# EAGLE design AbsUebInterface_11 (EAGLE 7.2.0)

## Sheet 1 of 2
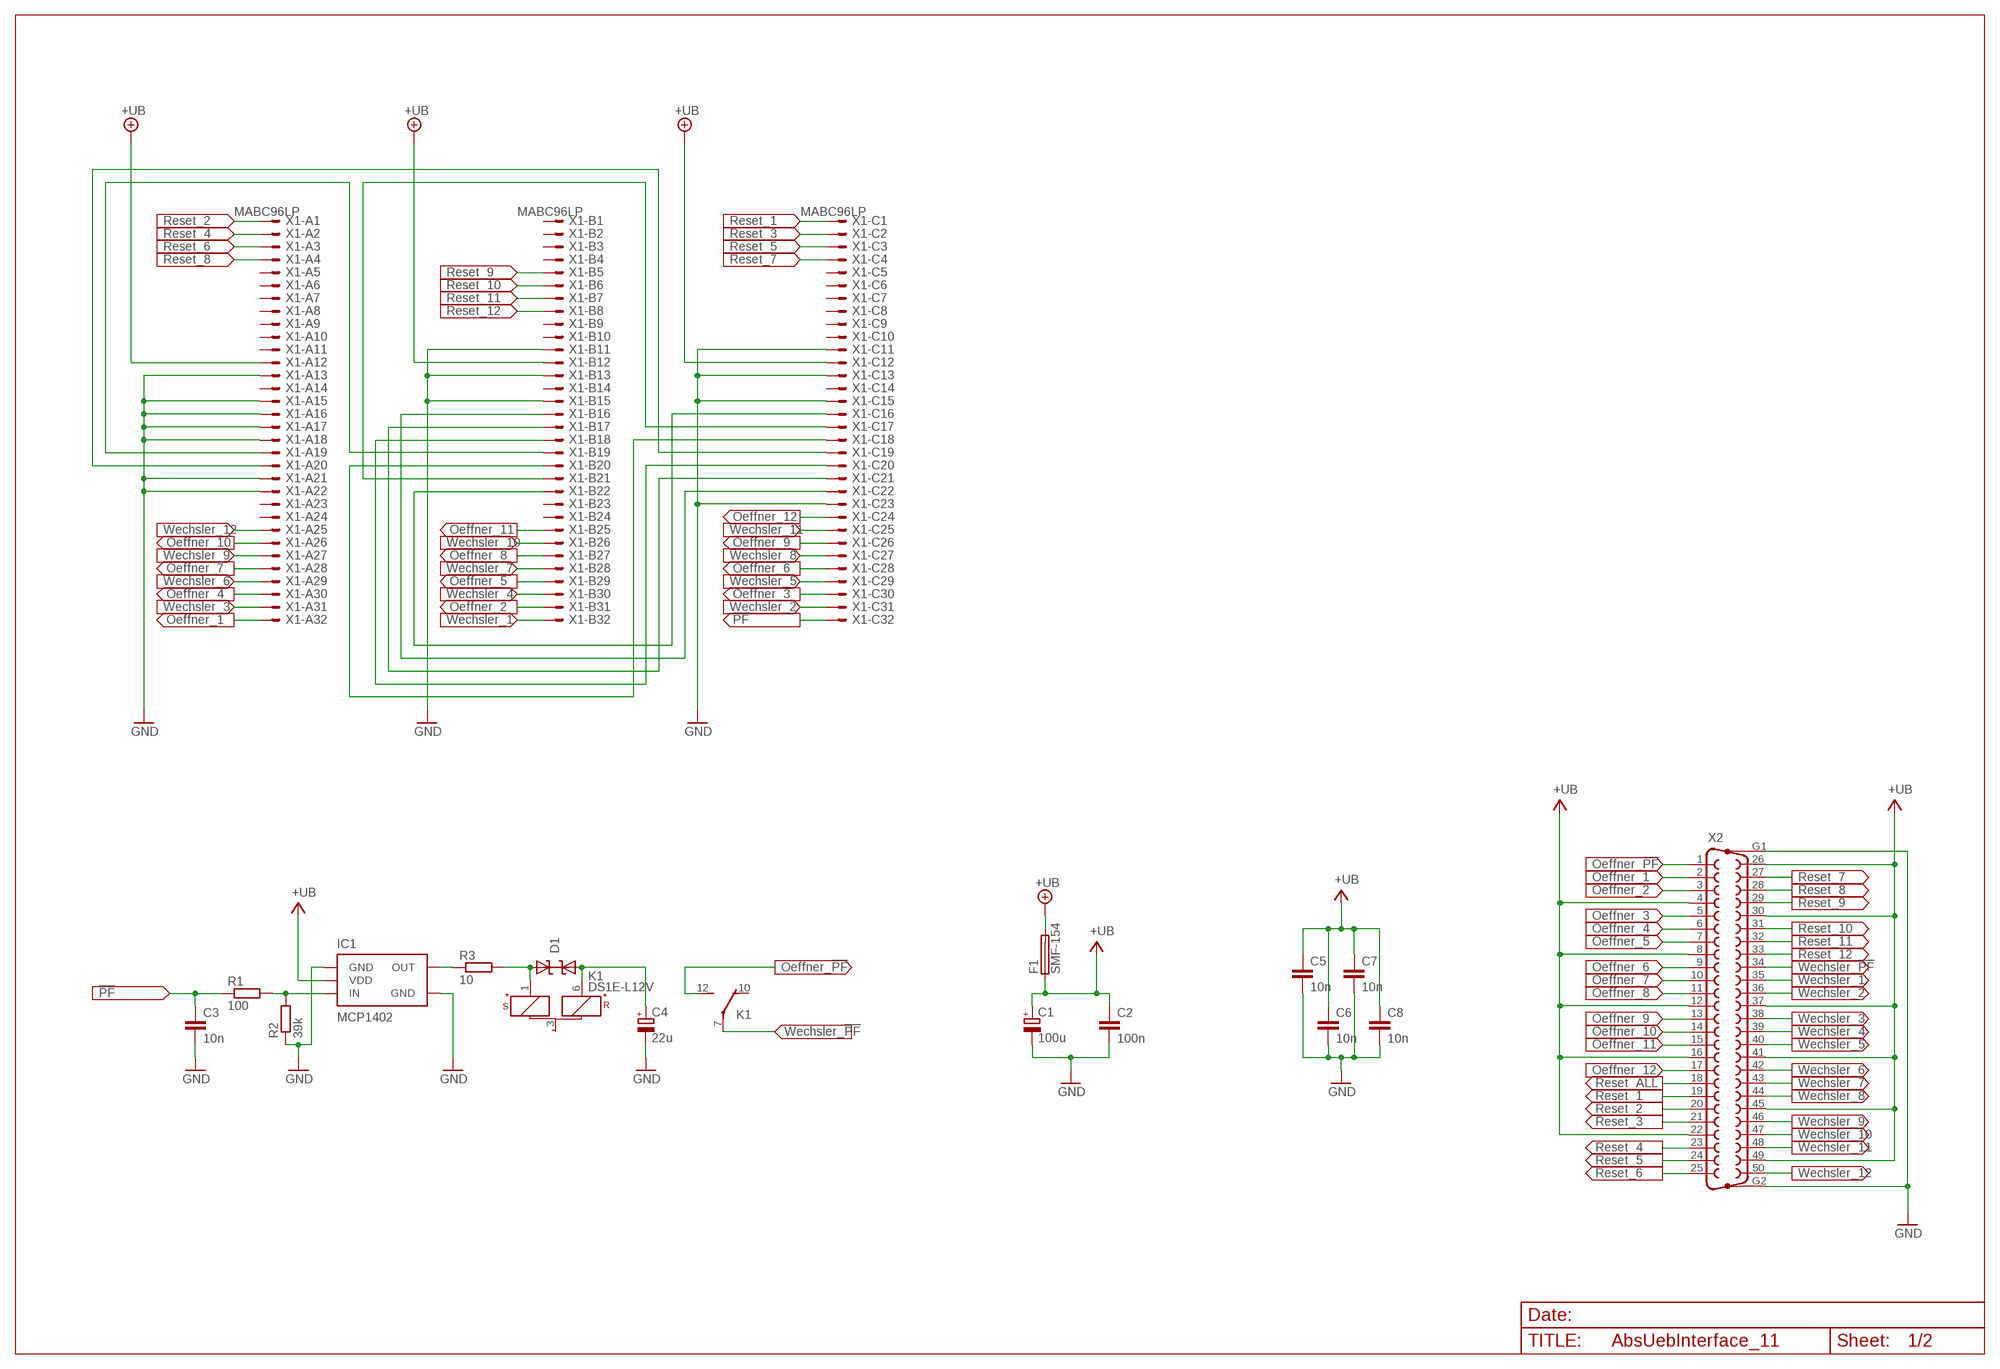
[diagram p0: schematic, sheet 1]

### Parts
C1  100u  CPOL-5-10  [RAD-FR-5,0-10]
C2  100n  C-SMD-1206  [C1206]
C3  10n  C-SMD-1206  [C1206]
C4  22u  CPOL-2-5  [RAD-FR-2,0-5]
C5  10n  C-SMD-1206  [C1206]
C6  10n  C-SMD-1206  [C1206]
C7  10n  C-SMD-1206  [C1206]
C8  10n  C-SMD-1206  [C1206]
D1  P6SMB11CAT3  [SMB-DO-214AA]
F1  SMF-154  [SMF-154]
IC1  MCP1402  [SOT223-5]
K1  DS1E-L12V  [DS1E-L]
R1  100  R-SMD-1206  [R1206]
R2  39k  R-SMD-1206  [R1206]
R3  10  R-SMD-1206  [R1206]
X1  MABC96LP  [MABC96LP]
X2  F50HP  [F50HP]

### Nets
1-WIRE: X1.B21 X1.C17
!PF: C3.1 R1.1 X1.C32
+UB: F1.2 X1.A12 X1.B12 X1.C12
CANH: X1.B16 X1.C22
CANL: X1.B22 X1.C16
EXT_PNP: X1.A20 X1.C19
EXT_RESET: X1.A19 X1.B19
GND: C1.- C2.2 C3.2 C4.- C5.2 C6.2 C7.2 C8.2 IC1.1(GND) IC1.4(GND) R2.1 X1.A13 X1.A15 X1.A16 X1.A17 X1.A18 X1.A21 X1.A22 X1.B11 X1.B13 X1.B15 X1.C11 X1.C13 X1.C15 X1.C23 X2.G1 X2.G2 ; also sheet 2
N$1: IC1.5(OUT) R3.1
N$2: D1.1(C) K1.1(1:S+) R3.2
N$3: IC1.3(IN) R1.2 R2.2
N$4: C4.+ D1.2(A) K1.6(1:R+)
N$5: X1.B20 X1.C18
OEFFNER_1: X1.A32 X2.2
OEFFNER_2: X1.B31 X2.3
OEFFNER_3: X1.C30 X2.5
OEFFNER_4: X1.A30 X2.6
OEFFNER_5: X1.B29 X2.7
OEFFNER_6: X1.C28 X2.9
OEFFNER_7: X1.A28 X2.10
OEFFNER_8: X1.B27 X2.11
OEFFNER_9: X1.C26 X2.13
OEFFNER_10: X1.A26 X2.14
OEFFNER_11: X1.B25 X2.15
OEFFNER_12: X1.C24 X2.17
OEFFNER_!PF: K1.12(2:S) X2.1
RESET_1: X1.C1 X2.19 ; also sheet 2
RESET_2: X1.A1 X2.20 ; also sheet 2
RESET_3: X1.C2 X2.21 ; also sheet 2
RESET_4: X1.A2 X2.23 ; also sheet 2
RESET_5: X1.C3 X2.24 ; also sheet 2
RESET_6: X1.A3 X2.25 ; also sheet 2
RESET_7: X1.C4 X2.27 ; also sheet 2
RESET_8: X1.A4 X2.28 ; also sheet 2
RESET_9: X1.B5 X2.29 ; also sheet 2
RESET_10: X1.B6 X2.31 ; also sheet 2
RESET_11: X1.B7 X2.32 ; also sheet 2
RESET_12: X1.B8 X2.33 ; also sheet 2
RESET_ALL: X2.18 ; also sheet 2
SCL: X1.B18 X1.C20
SDA: X1.B17 X1.C21
V+: C1.+ C2.1 C5.1 C6.1 C7.1 C8.1 F1.1 IC1.2(VDD) X2.4 X2.8 X2.12 X2.16 X2.22 X2.26 X2.30 X2.37 X2.41 X2.45 X2.49 ; supply symbol labelled +UB ; also sheet 2
WECHSLER_1: X1.B32 X2.35
WECHSLER_2: X1.C31 X2.36
WECHSLER_3: X1.A31 X2.38
WECHSLER_4: X1.B30 X2.39
WECHSLER_5: X1.C29 X2.40
WECHSLER_6: X1.A29 X2.42
WECHSLER_7: X1.B28 X2.43
WECHSLER_8: X1.C27 X2.44
WECHSLER_9: X1.A27 X2.46
WECHSLER_10: X1.B26 X2.47
WECHSLER_11: X1.C25 X2.48
WECHSLER_12: X1.A25 X2.50
WECHSLER_!PF: K1.7(2:P) X2.34
Unconnected: K1.3(1:-) K1.10(2:O) X1.A5 X1.A6 X1.A7 X1.A8 X1.A9 X1.A10 X1.A11 X1.A14 X1.A23 X1.A24 X1.B1 X1.B2 X1.B3 X1.B4 X1.B9 X1.B10 X1.B14 X1.B23 X1.B24 X1.C5 X1.C6 X1.C7 X1.C8 X1.C9 X1.C10 X1.C14

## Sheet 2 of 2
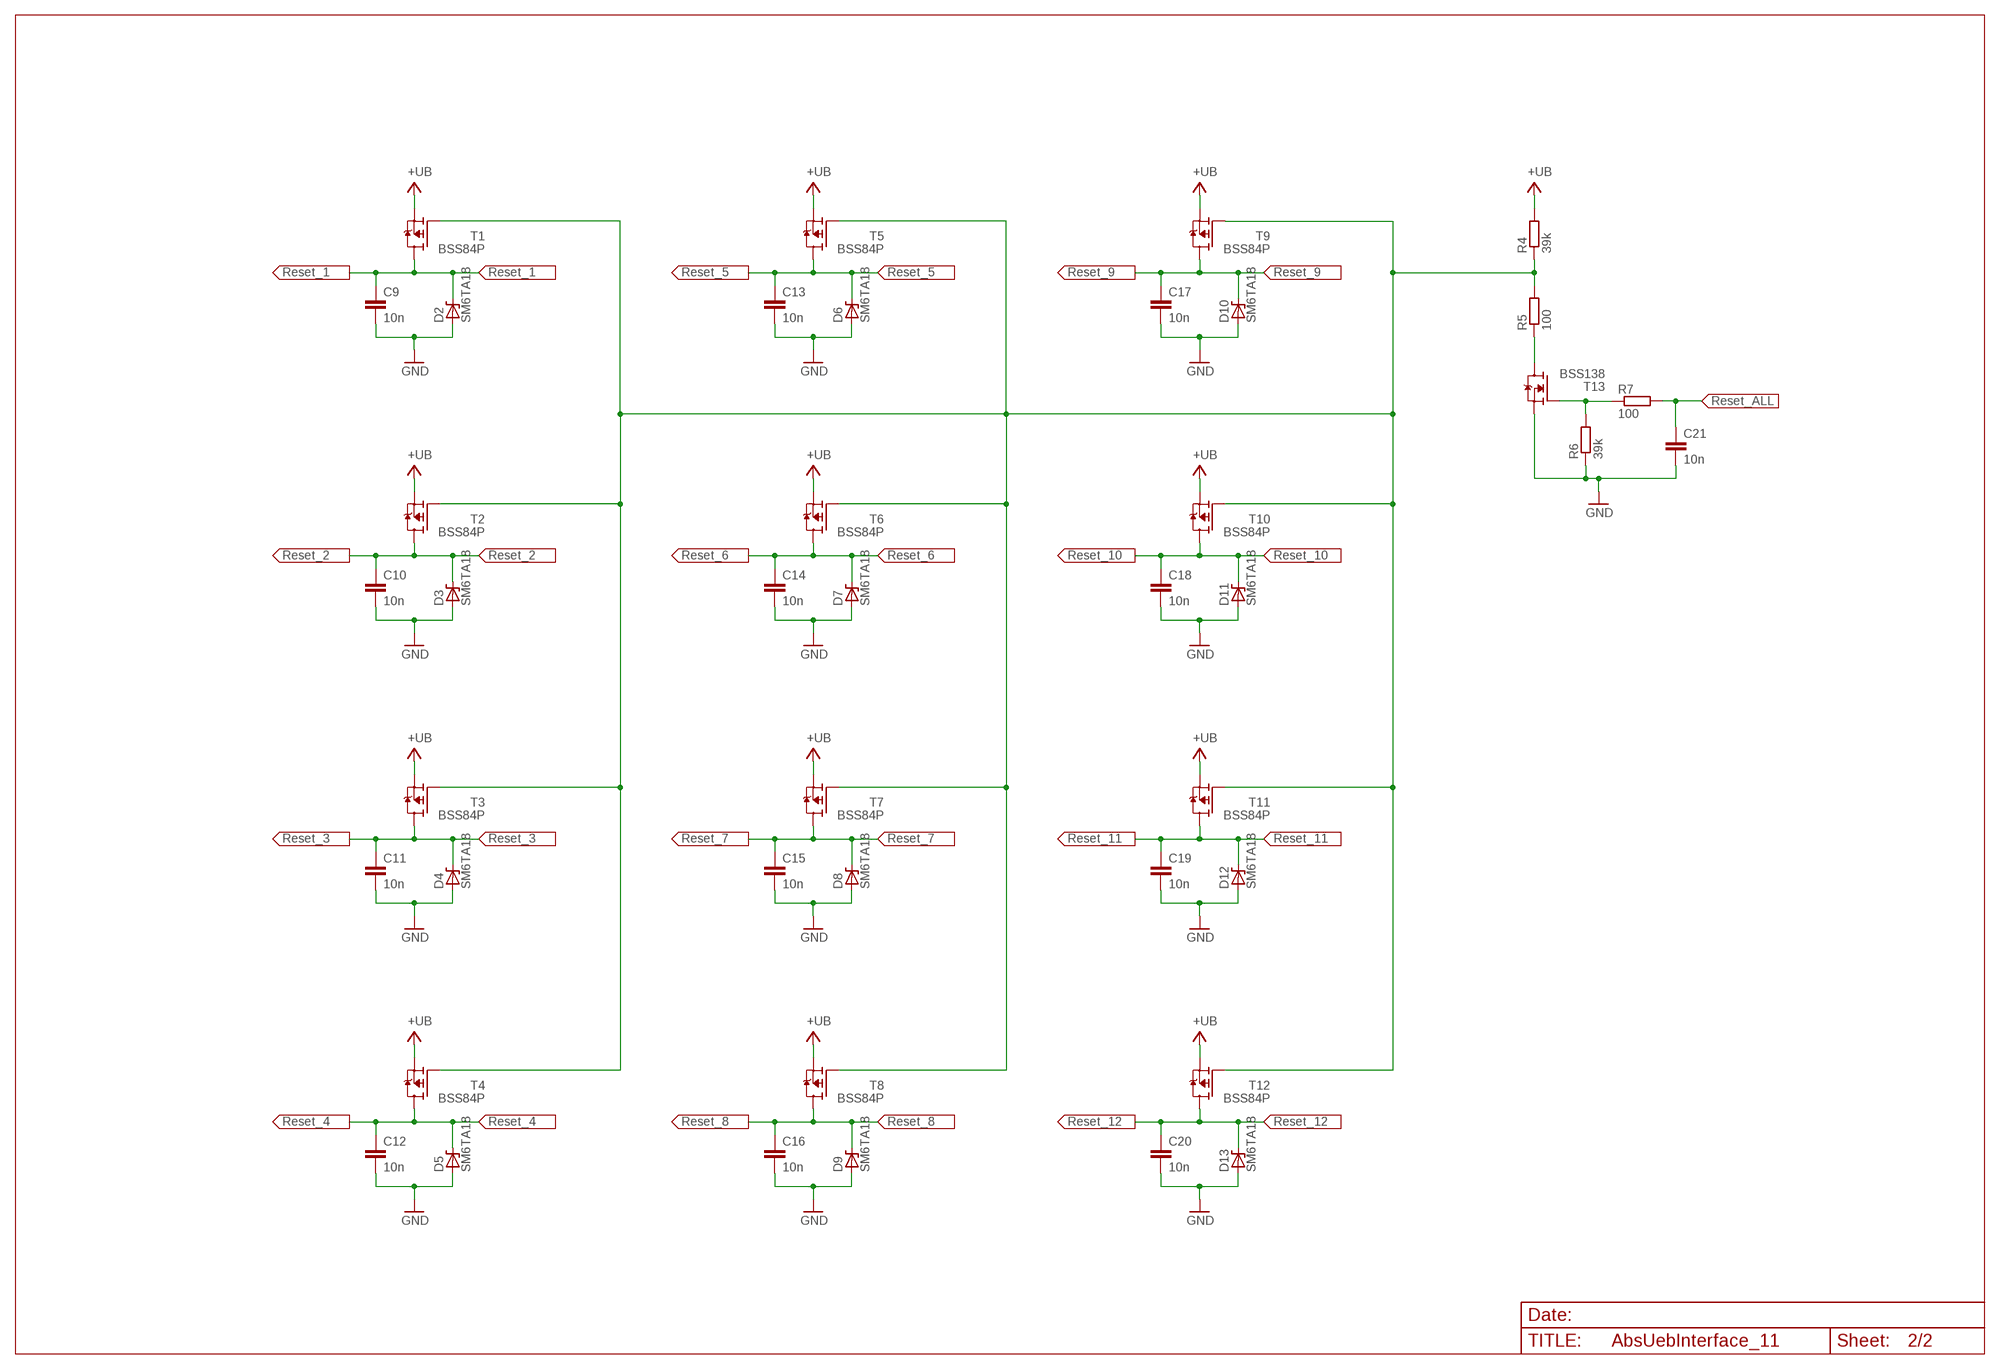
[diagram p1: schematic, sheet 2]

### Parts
C9  10n  C-SMD-1206  [C1206]
C10  10n  C-SMD-1206  [C1206]
C11  10n  C-SMD-1206  [C1206]
C12  10n  C-SMD-1206  [C1206]
C13  10n  C-SMD-1206  [C1206]
C14  10n  C-SMD-1206  [C1206]
C15  10n  C-SMD-1206  [C1206]
C16  10n  C-SMD-1206  [C1206]
C17  10n  C-SMD-1206  [C1206]
C18  10n  C-SMD-1206  [C1206]
C19  10n  C-SMD-1206  [C1206]
C20  10n  C-SMD-1206  [C1206]
C21  10n  C-SMD-1206  [C1206]
D2  SM6TA18  [DO-214AA]
D3  SM6TA18  [DO-214AA]
D4  SM6TA18  [DO-214AA]
D5  SM6TA18  [DO-214AA]
D6  SM6TA18  [DO-214AA]
D7  SM6TA18  [DO-214AA]
D8  SM6TA18  [DO-214AA]
D9  SM6TA18  [DO-214AA]
D10  SM6TA18  [DO-214AA]
D11  SM6TA18  [DO-214AA]
D12  SM6TA18  [DO-214AA]
D13  SM6TA18  [DO-214AA]
R4  39k  R-SMD-1206  [R1206]
R5  100  R-SMD-1206  [R1206]
R6  39k  R-SMD-1206  [R1206]
R7  100  R-SMD-1206  [R1206]
T1  BSS84P  [SOT23]
T2  BSS84P  [SOT23]
T3  BSS84P  [SOT23]
T4  BSS84P  [SOT23]
T5  BSS84P  [SOT23]
T6  BSS84P  [SOT23]
T7  BSS84P  [SOT23]
T8  BSS84P  [SOT23]
T9  BSS84P  [SOT23]
T10  BSS84P  [SOT23]
T11  BSS84P  [SOT23]
T12  BSS84P  [SOT23]
T13  BSS138  [SOT23]

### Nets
GND: C9.2 C10.2 C11.2 C12.2 C13.2 C14.2 C15.2 C16.2 C17.2 C18.2 C19.2 C20.2 C21.2 D2.1(A) D3.1(A) D4.1(A) D5.1(A) D6.1(A) D7.1(A) D8.1(A) D9.1(A) D10.1(A) D11.1(A) D12.1(A) D13.1(A) R6.1 T13.2(S) ; also sheet 1
N$6: R6.2 R7.1 T13.1(G)
N$7: R5.1 T13.3(D)
N$8: R4.1 R5.2 T1.1(G) T2.1(G) T3.1(G) T4.1(G) T5.1(G) T6.1(G) T7.1(G) T8.1(G) T9.1(G) T10.1(G) T11.1(G) T12.1(G)
RESET_1: C9.1 D2.2(C) T1.3(D) ; also sheet 1
RESET_2: C10.1 D3.2(C) T2.3(D) ; also sheet 1
RESET_3: C11.1 D4.2(C) T3.3(D) ; also sheet 1
RESET_4: C12.1 D5.2(C) T4.3(D) ; also sheet 1
RESET_5: C13.1 D6.2(C) T5.3(D) ; also sheet 1
RESET_6: C14.1 D7.2(C) T6.3(D) ; also sheet 1
RESET_7: C15.1 D8.2(C) T7.3(D) ; also sheet 1
RESET_8: C16.1 D9.2(C) T8.3(D) ; also sheet 1
RESET_9: C17.1 D10.2(C) T9.3(D) ; also sheet 1
RESET_10: C18.1 D11.2(C) T10.3(D) ; also sheet 1
RESET_11: C19.1 D12.2(C) T11.3(D) ; also sheet 1
RESET_12: C20.1 D13.2(C) T12.3(D) ; also sheet 1
RESET_ALL: C21.1 R7.2 ; also sheet 1
V+: R4.2 T1.2(S) T2.2(S) T3.2(S) T4.2(S) T5.2(S) T6.2(S) T7.2(S) T8.2(S) T9.2(S) T10.2(S) T11.2(S) T12.2(S) ; supply symbol labelled +UB ; also sheet 1

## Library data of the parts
C1 = AbsUebParts_11:CPOL-5-10: Elektrolytkondensator RM 5,0mm; MF: Panasonic; OC_REICHELT: RAD FR 100/63
C2 C3 C5-C21 = AbsUebParts_11:C-SMD: SMD Keramik Vielschichtkondensatoren
C4 = AbsUebParts_11:CPOL-2-5: Elektrolytkondensator RM 2,0mm; MF: Panasonic; OC_REICHELT: RAD FR 22/50
D1 = AbsUebParts_11:P6SMB11CAT3: Suppressor diode bi-directional
D2-D13 = AbsUebParts_11:SM6TA: STM Transil Suppressor Diode; MF: STM; MPN: SM6T18A; OC_REICHELT: P6SMB 18A SMD
F1 = AbsUebParts_11:SMF-154: Littelfuse Surface Mount Fuse; MF: Littelfuse; MPN: 154.250; OC_REICHELT: SMD-HASF 0,25A; OC_RS: 219-6068
IC1 = AbsUebParts_11:MCP1402: MCP1402 500mA. High-Speed Power MOSFET Driver; MF: Microchip; MPN: MCP1402; OC_RS: 668-4203
K1 = AbsUebParts_11:DS1E-L*: DS-RELAYS HIGHLY SENSITIVE 1500 V FCC SURGE NAiS WITHSTANDING MINIATURE RELAY Source: http://www.mew-europe.com/.. en_ds_61005_0001.pdf; MF: Panasonic; MPN: DS2E-SL2-DC12V; OC_RS: 815-4988
R1-R7 = AbsUebParts_11:R-SMD: SMD Resistor
T1-T12 = AbsUebParts_11:BSS84P: Infineon SIPMOS P-Channel Small-Signal-Transistor; MF: Infineon; MPN: BSS 84 P; OC_REICHELT: BSS 84P SMD
T13 = AbsUebParts_11:BSS138: Infineon NFET N-Channel Logic Level Enhancement Mode Field Effect Transistor; MF: FSC; MPN: BSS138; OC_REICHELT: BSS 138 SMD
X1 = AbsUebParts_11:MABC96LP: CONNECTOR male, 96 pins, type C, rows ABC, grid 2.54 mm with mounting clip; MF: ept; OC_REICHELT: ML-C 96W
X2 = AbsUebParts_11:F50HP: SUB-D; MF: CONEC; MPN: 164A18759X; OC_FARNELL: unknown; OC_REICHELT: D-SUB BU 50GWC

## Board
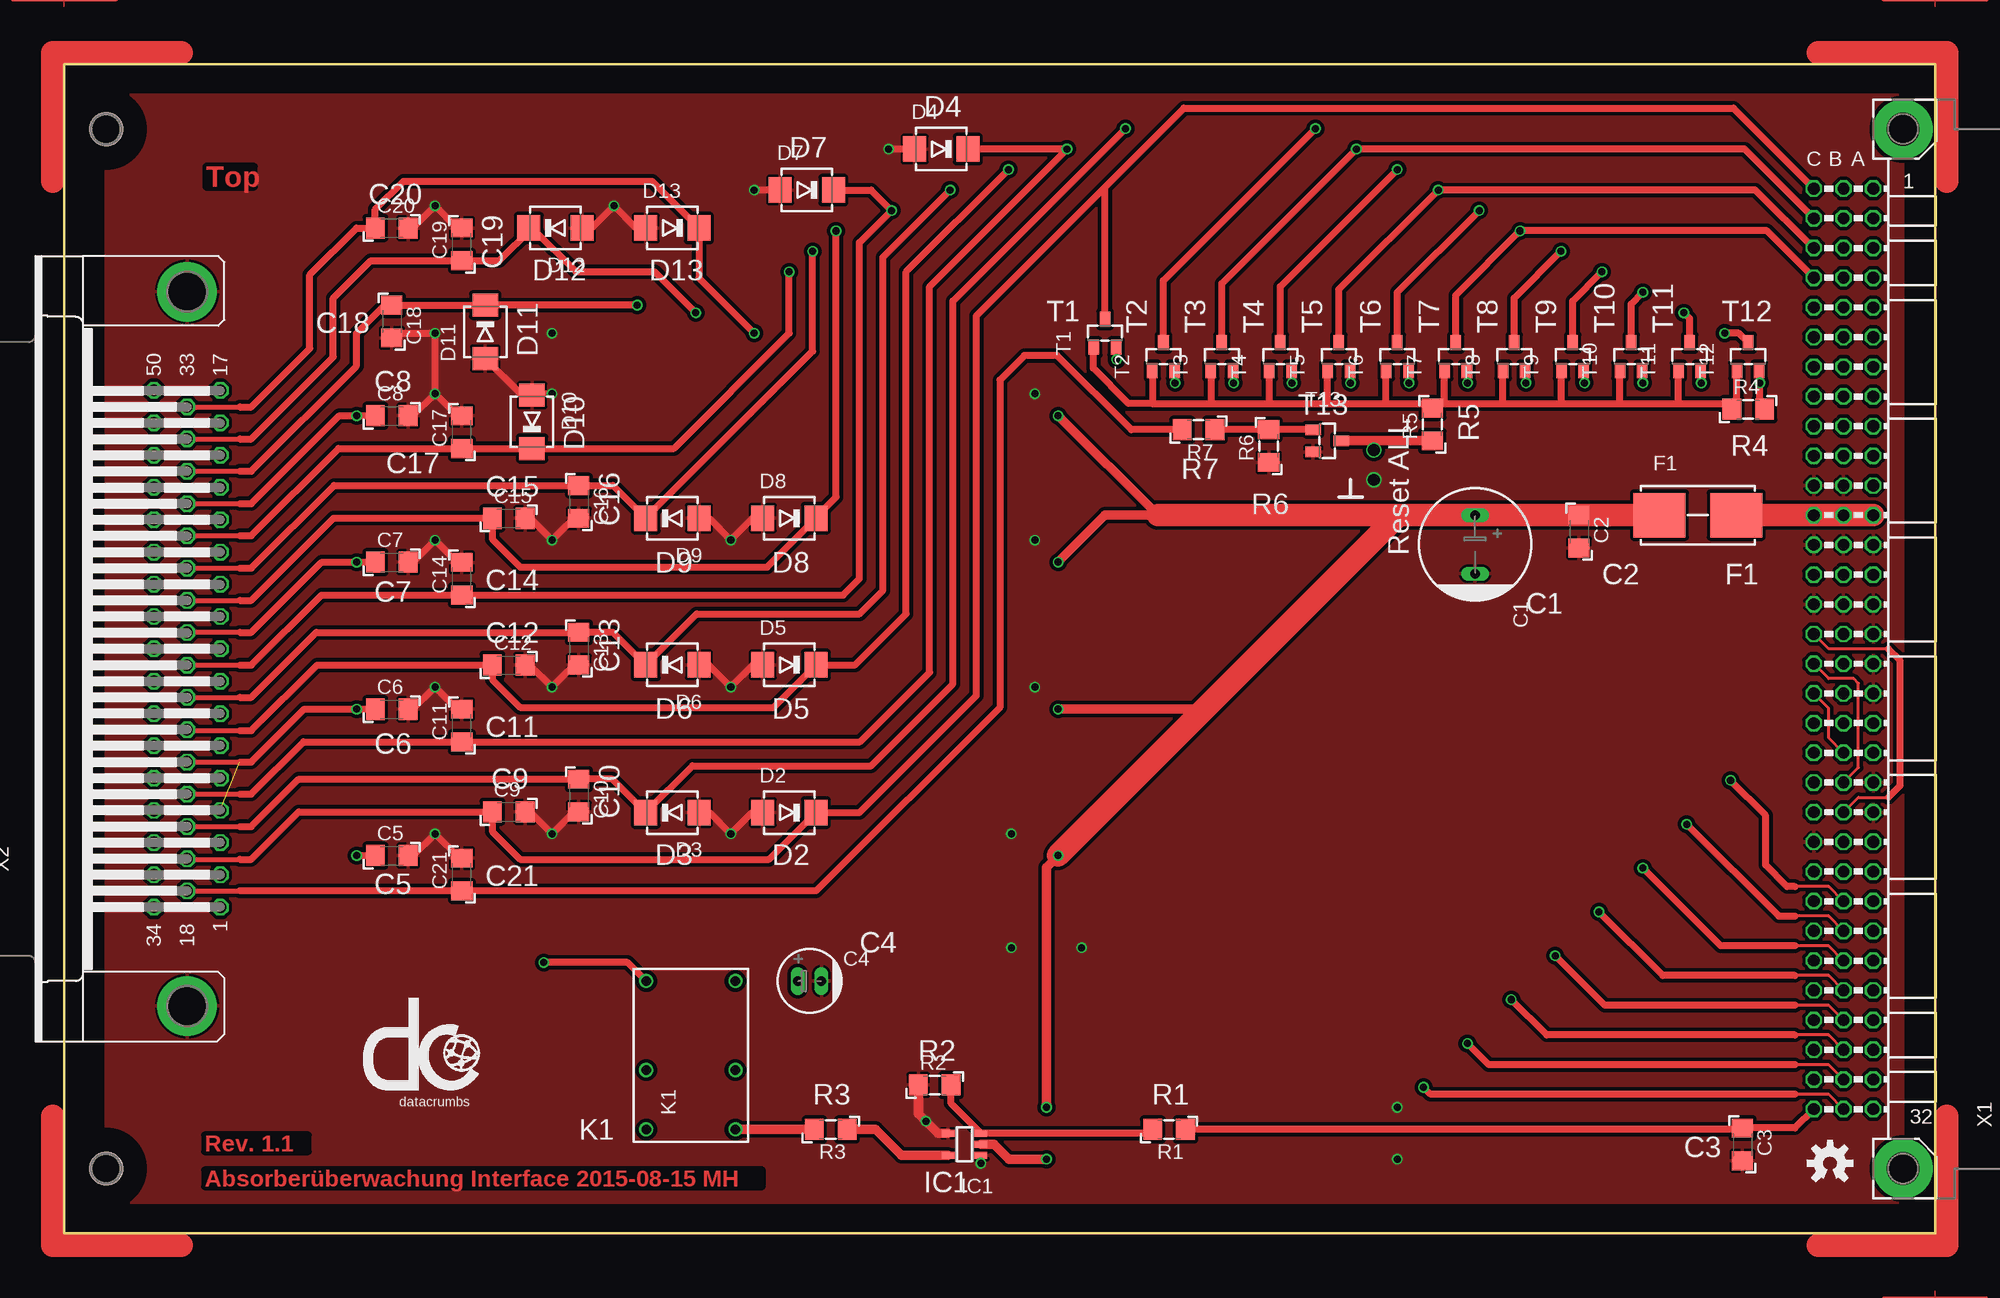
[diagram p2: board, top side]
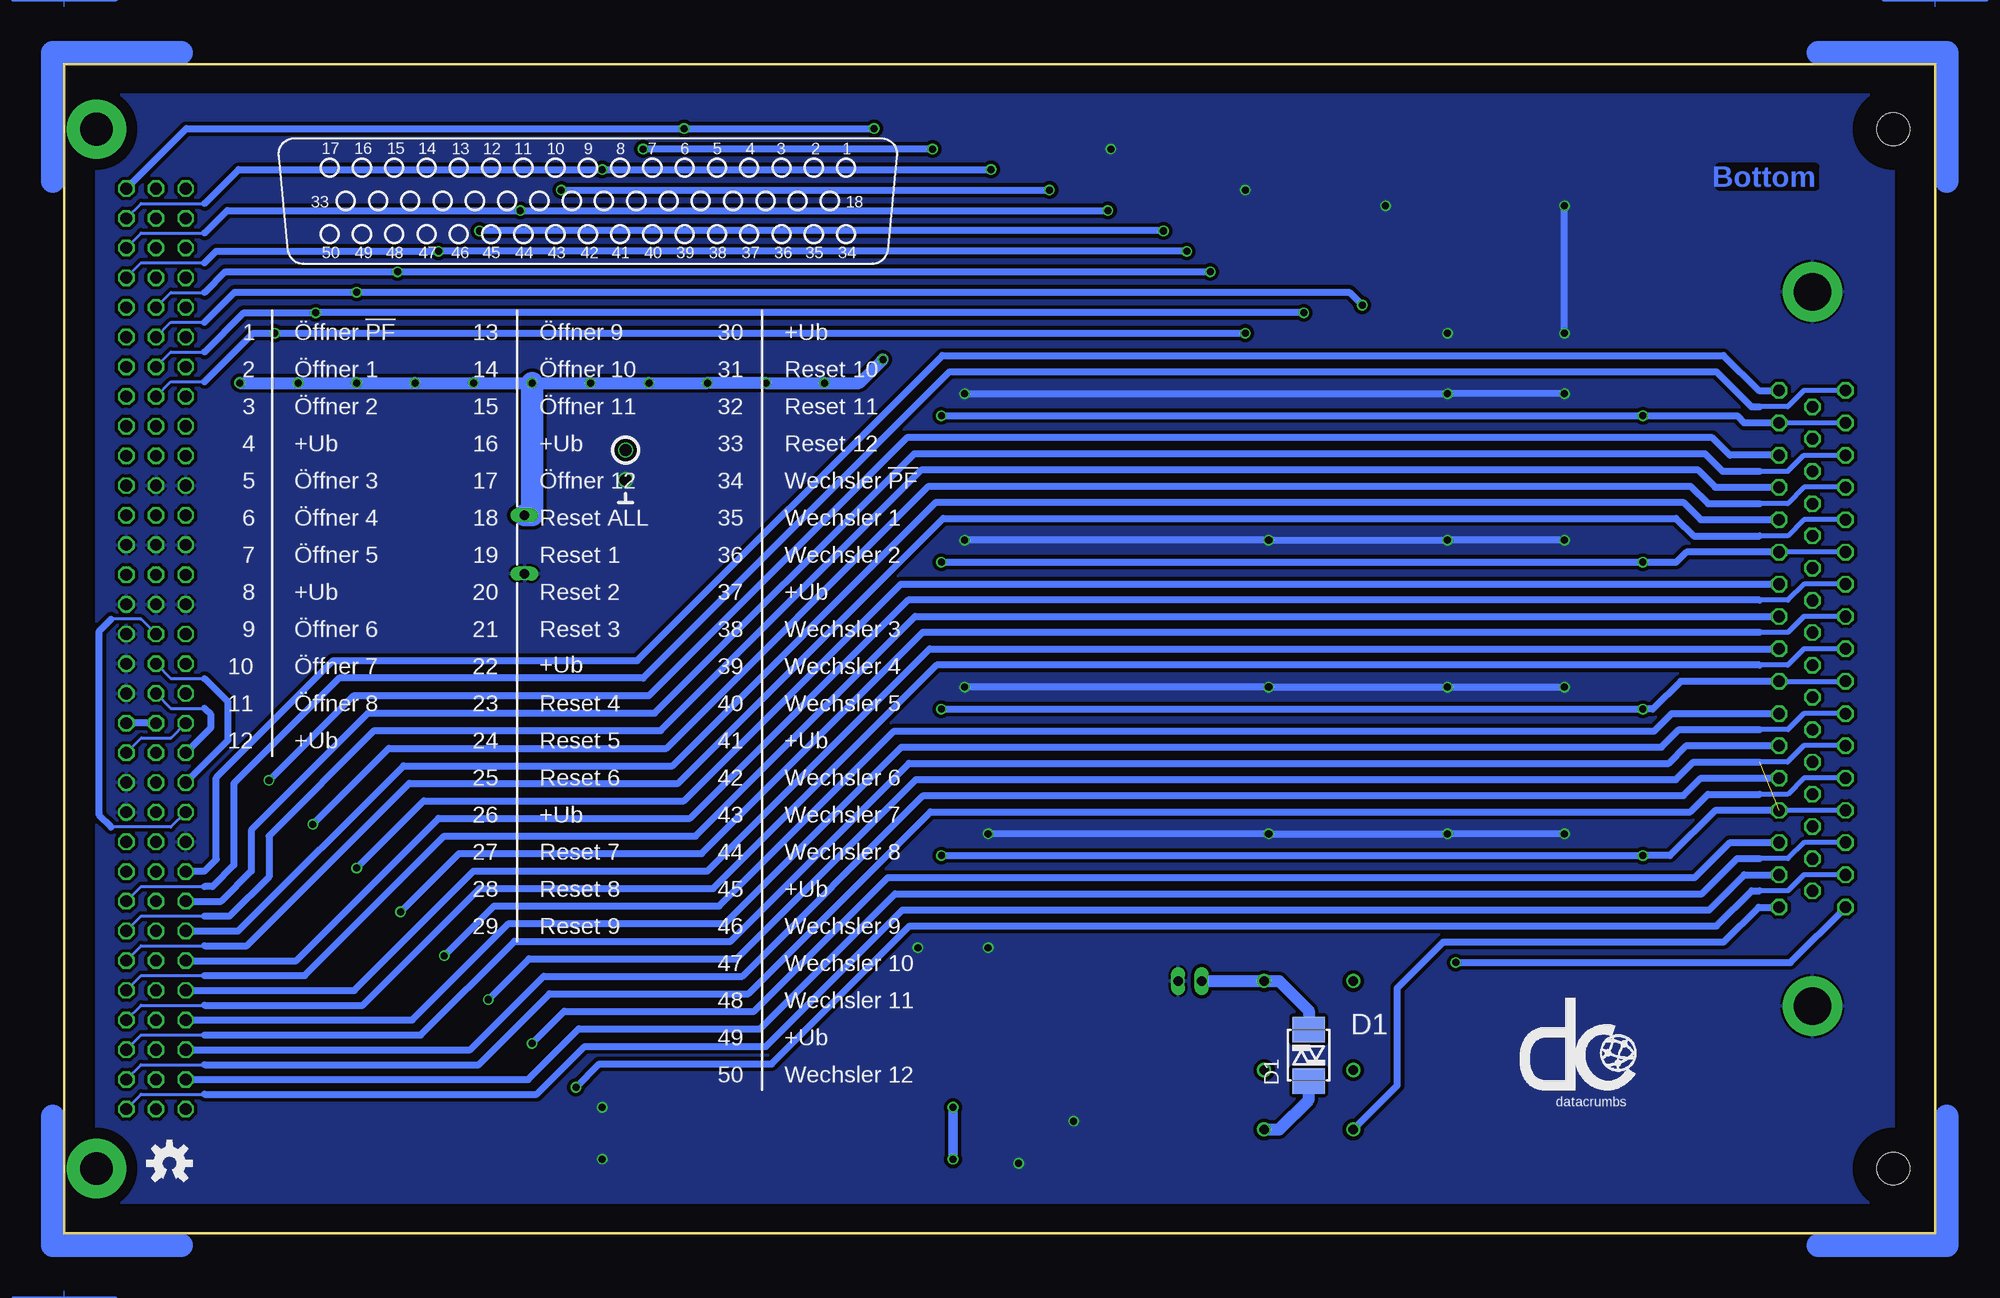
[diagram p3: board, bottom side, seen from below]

Size 160.03 x 100.03 mm. Coordinates in mm from the lower left corner, seen from the top.
Outline: 0,0.01 160,0.01 160,100.01 0,100.01 0,0.01
Copper layers (1*16): Top 0.035mm / dielectric 1.5mm / Bottom 0.035mm
Design rules "Aetzwerk-DRC 2 Lagen 35µm Cu *": minimum track width 6mil, minimum drill 12mil, track to track 6mil, track to pad 6mil, pad to pad 6mil, via to via 6mil, smd to smd 6mil, copper to edge 20mil, drill to drill 8mil, minimum pad ring 8mil, minimum via ring 6mil, stop-mask expansion 3mil, vias tented up to drill 24mil, thermal gap 8mil
Holes 2.8 mm at 3.57,94.46 3.57,5.56
tKeepout: area 0,0 to 160,2.5; area 0,97.5 to 160,100
bKeepout: area 0,0 to 160,2.5; area 0,97.5 to 160,100
tRestrict: area 1.3,92.2 to 5.9,96.7; area 1.3,3.3 to 5.9,7.8
bRestrict: area 1.3,92.2 to 5.9,96.7; area 1.3,3.3 to 5.9,7.8
vRestrict: area 1.3,3.3 to 5.9,7.8; area 1.3,92.2 to 5.9,96.7

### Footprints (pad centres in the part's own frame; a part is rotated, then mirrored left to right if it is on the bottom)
RAD-FR-5,0-10 = drill 0.8 long: + -2.5,0; - 2.5,0
C1206 = smd 1.6 x 1.8: 1 -1.4,0; 2 1.4,0
RAD-FR-2,0-5 = drill 0.8 long: + -1,0; - 1,0
SMB-DO-214AA = smd 2.16 x 2.75: 1 -2.2,0; 2 2.2,0
DO-214AA = smd 1.96 x 2.18: 1 -2.28,0; 2 2.28,0
SMF-154 = smd 4.445 x 3.81: 1 -3.289,0; 2 3.289,0
SOT223-5 = smd 0.6 x 1.1: 1 -0.95,-1.4; 2 0,-1.4; 3 0.95,-1.4; 4 0.95,1.4; 5 -0.95,1.4
DS1E-L = drill 0.8: 1 -6.35,-3.81; 3 -1.27,-3.81; 6 6.35,-3.81; 7 6.35,3.81; 10 -1.27,3.81; 12 -6.35,3.81
R1206 = smd 1.6 x 1.8: 1 -1.4,0; 2 1.4,0
SOT23 = smd 0.9 x 1.3: 1 -0.95,-1.2; 2 0.95,-1.2; 3 0,1.2
MABC96LP = drill 1 octagon: A1 -2.54,39.37; A2 -2.54,36.83; A3 -2.54,34.29; A4 -2.54,31.75; A5 -2.54,29.21; A6 -2.54,26.67; A7 -2.54,24.13; A8 -2.54,21.59; A9 -2.54,19.05; A10 -2.54,16.51; A11 -2.54,13.97; A12 -2.54,11.43; A13 -2.54,8.89; A14 -2.54,6.35; A15 -2.54,3.81; A16 -2.54,1.27; A17 -2.54,-1.27; A18 -2.54,-3.81; A19 -2.54,-6.35; A20 -2.54,-8.89; A21 -2.54,-11.43; A22 -2.54,-13.97; A23 -2.54,-16.51; A24 -2.54,-19.05; A25 -2.54,-21.59; A26 -2.54,-24.13; A27 -2.54,-26.67; A28 -2.54,-29.21; A29 -2.54,-31.75; A30 -2.54,-34.29; A31 -2.54,-36.83; A32 -2.54,-39.37; B1 -5.08,39.37; B2 -5.08,36.83; B3 -5.08,34.29; B4 -5.08,31.75; B5 -5.08,29.21; B6 -5.08,26.67; B7 -5.08,24.13; B8 -5.08,21.59; B9 -5.08,19.05; B10 -5.08,16.51; B11 -5.08,13.97; B12 -5.08,11.43; B13 -5.08,8.89; B14 -5.08,6.35; B15 -5.08,3.81; B16 -5.08,1.27; B17 -5.08,-1.27; B18 -5.08,-3.81; B19 -5.08,-6.35; B20 -5.08,-8.89; B21 -5.08,-11.43; B22 -5.08,-13.97; B23 -5.08,-16.51; B24 -5.08,-19.05; B25 -5.08,-21.59; B26 -5.08,-24.13; B27 -5.08,-26.67; B28 -5.08,-29.21; B29 -5.08,-31.75; B30 -5.08,-34.29; B31 -5.08,-36.83; B32 -5.08,-39.37; C1 -7.62,39.37; C2 -7.62,36.83; C3 -7.62,34.29; C4 -7.62,31.75; C5 -7.62,29.21; C6 -7.62,26.67; C7 -7.62,24.13; C8 -7.62,21.59; C9 -7.62,19.05; C10 -7.62,16.51; C11 -7.62,13.97; C12 -7.62,11.43; C13 -7.62,8.89; C14 -7.62,6.35; C15 -7.62,3.81; C16 -7.62,1.27; C17 -7.62,-1.27; C18 -7.62,-3.81; C19 -7.62,-6.35; C20 -7.62,-8.89; C21 -7.62,-11.43; C22 -7.62,-13.97; C23 -7.62,-16.51; C24 -7.62,-19.05; C25 -7.62,-21.59; C26 -7.62,-24.13; C27 -7.62,-26.67; C28 -7.62,-29.21; C29 -7.62,-31.75; C30 -7.62,-34.29; C31 -7.62,-36.83; C32 -7.62,-39.37 | drill 2.8 pad 5.08: X1 0,44.45; X2 0,-44.45
F50HP = drill 1 octagon: 1 -22.1,-2.84; 2 -19.33,-2.84; 3 -16.56,-2.84; 4 -13.82,-2.84; 5 -11.05,-2.84; 6 -8.28,-2.84; 7 -5.54,-2.84; 8 -2.77,-2.84; 9 0,-2.84; 10 2.77,-2.84; 11 5.54,-2.84; 12 8.28,-2.84; 13 11.05,-2.84; 14 13.82,-2.84; 15 16.56,-2.84; 16 19.33,-2.84; 17 22.1,-2.84; 18 -20.7,0; 19 -17.96,0; 20 -15.19,0; 21 -12.42,0; 22 -9.68,0; 23 -6.91,0; 24 -4.14,0; 25 -1.4,0; 26 1.4,0; 27 4.14,0; 28 6.91,0; 29 9.68,0; 30 12.42,0; 31 15.19,0; 32 17.96,0; 33 20.7,0; 34 -22.1,2.84; 35 -19.33,2.84; 36 -16.56,2.84; 37 -13.82,2.84; 38 -11.05,2.84; 39 -8.28,2.84; 40 -5.54,2.84; 41 -2.77,2.84; 42 0,2.84; 43 2.77,2.84; 44 5.54,2.84; 45 8.28,2.84; 46 11.05,2.84; 47 13.82,2.84; 48 16.56,2.84; 49 19.33,2.84; 50 22.1,2.84 | drill 3.2 pad 5.08: G1 -30.55,0; G2 30.55,0

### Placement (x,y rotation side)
C1  120.65,58.94 270 top
C2  129.54,60.04 270 top
C3  143.51,7.63 270 top
C4  63.74,21.6 0 top
C5  28,32.33 0 top
C6  28,44.85 0 top
C7  28,57.42 0 top
C8  28,69.95 0 top
C9  38,36.07 0 top
C10  44,37.47 270 top
C11  34,43.45 90 top
C12  38,48.63 0 top
C13  44,50.03 270 top
C14  34,56.01 90 top
C15  38,61.18 0 top
C16  44,62.58 270 top
C17  34,68.55 90 top
C18  28,78.01 270 top
C19  34,84.61 90 top
C20  28,86.01 0 top
C21  34,30.71 90 top
D1  53.58,15.25 90 bottom
D2  62,36.01 0 top
D3  52,36.01 180 top
D4  75,92.76 0 top
D5  62,48.64 0 top
D6  52,48.64 180 top
D7  63.5,89.26 0 top
D8  62,61.18 0 top
D9  52,61.18 180 top
D10  40,69.43 270 top
D11  36,77.13 90 top
D12  42,86.01 180 top
D13  52,86.01 0 top
DRILEGEND  [DRILEGEND]  not placed on the board
F1  139.7,61.44 0 top
IC1  76.98,7.63 90 top
K1  53.58,15.25 90 top
PM1  [PASSMARK]  not placed on the board
PM2  [PASSMARK]  not placed on the board
PM3  [PASSMARK]  not placed on the board
R1  94.47,8.9 180 top
R2  74.44,12.71 0 top
R3  65.55,8.9 180 top
R4  144,70.51 0 top
R5  117,69.21 90 top
R6  103,67.36 90 top
R7  97,68.76 180 top
T1  89,77.01 0 top
T2  94,75.01 0 top
T3  99,75.01 0 top
T4  104,75.01 0 top
T5  109,75.01 0 top
T6  114,75.01 0 top
T7  119,75.01 0 top
T8  124,75.01 0 top
T9  129,75.01 0 top
T10  134,75.01 0 top
T11  139,75.01 0 top
T12  144,75.01 0 top
T13  108,67.81 270 top
X1  157.24,50.01 0 top
X2  10.5,50.01 90 top

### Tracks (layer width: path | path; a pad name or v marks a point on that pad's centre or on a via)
1-WIRE
  Top 0.254: X1.B21 153.44,39.86 153.44,47.06 153.02,47.47 150.89,47.47 X1.C17
!PF
  Top 0.61: X1.C32 148.01,9.03 C3.1 143.38,8.9 R1.1
+UB
  Top 1.93: F1.2 X1.C12 X1.B12 X1.A12
CANH
  Bottom 0.254: X1.C22 150.89,34.77 156,34.77 | X1.B16 153.43,52.55 156,52.55
  Bottom 0.61: 156,34.77 157,35.77 157,51.55 156,52.55
CANL
  Top 0.254: X1.B22 153.43,37.31 156,37.31 | 156,50.01 150.89,50.01 X1.C16
  Top 0.61: 156,37.31 157,38.31 157,49.01 156,50.01
CM10
  Top 2: -1,10.01 -1,-0.99 10,-0.99
CM11
  Bottom 2: 10,-0.99 -1,-0.99 -1,10.01
CM20
  Top 2: 150,-0.99 161,-0.99 161,10.01
CM21
  Bottom 2: 150,-0.99 161,-0.99 161,10.01
CM30
  Top 2: 10,101.01 -1,101.01 -1,90.01
CM31
  Bottom 2: -1,90.01 -1,101.01 10,101.01
CM40
  Top 2: 150,101.01 161,101.01 161,90.01
CM41
  Bottom 2: 150,101.01 161,101.01 161,90.01
EXT_PNP
  Bottom 0.254: X1.A20 153.42,42.41 150.88,42.41 X1.C19
EXT_RESET
  Bottom 0.61: X1.B19 X1.A19
GND  (via drill 0.6, 1)
  Top 0.406: v78.38,6.01 IC1.1
  Top 0.61: C15.2 39.82,61.18 v41.7,59.3 43.58,61.18 C16.2 | C12.2 39.81,48.63 v41.7,46.74 43.59,48.63 C13.2 | C9.2 39.83,36.07 v41.7,34.2 43.57,36.07 C10.2 44.06,36.01 | C8.2 29.81,69.95 v31.7,71.84 | C17.2 33.59,69.95 v31.7,71.84 | C7.2 29.82,57.42 v31.7,59.3 33.59,57.41 C14.2 | C6.2 29.81,44.85 v31.7,46.74 33.59,44.85 C11.2 | C19.2 33.59,86.01 v31.7,87.9 29.81,86.01 C20.2 | v31.7,71.84 v31.7,77.01 28.4,77.01 C18.2 | 39.87,71.84 D10.1 40.13,71.84 v41.7,71.84 39.01,71.84 D11.1 | D3.1 55.19,36.01 v57,34.2 58.81,36.01 D2.1 | D6.1 55.1,48.64 v57,46.74 58.9,48.64 D5.1 | D9.1 55.12,61.18 v57,59.3 58.88,61.18 D8.1 | D13.1 48.89,86.01 v47,87.9 45.11,86.01 D12.1 | D7.1 v59,89.26 | D4.1 v70.5,92.76 | 33.79,32.11 v31.7,34.2 29.83,32.33 C5.2
  Top 0.813: IC1.4 74.71,8.58 v73.67,9.61 73.04,10.25 R2.1
  Bottom 0.61: v31.7,34.2 v41.7,34.2 v57,34.2 v81,34.2 | v31.7,59.3 v41.7,59.3 v57,59.3 v83,59.3 | v31.7,46.74 v41.7,46.74 v57,46.74 v83,46.74 | v31.7,77.01 v31.7,87.9 | v31.7,71.84 v41.7,71.84 v83,71.84
  other vias: 114,10.8 114,6.36 81,24.44 41.7,77.01 87,24.44 112,64.47
  pour Top (isolate 0.305): 3.57,2.66 157.24,2.66 157.24,97.36 3.57,97.36
  pour Bottom (isolate 0.305): 3.57,2.66 157.24,2.66 157.24,97.36 3.57,97.36
N$1
  Top 0.813: IC1.5 71.58,6.68 69.36,8.9 R3.1
N$2
  Top 0.813: K1.1 R3.2
  Bottom 1.016: K1.1 56.12,8.9 53.58,11.44 D1.1
N$3
  Top 0.61: R1.2 92.75,8.58 IC1.3 75.84,11.12 R2.2
N$4
  Bottom 1.016: C4.+ K1.6 56.12,21.6 53.58,19.06 D1.2
N$5
  Top 0.254: X1.B20 150.89,42.39 150.89,44.93 X1.C18
N$6
  Top 0.61: T13.1 R6.2 R7.1
N$7  (via drill 1)
  Top 0.813: T13.3 112,67.81 | 112,67.81 R5.1 | v112,67.01 112,67.81
N$8
  Top 0.61: 93,71.01 98,71.01 | 108,71.01 113,71.01 | 118,71.01 123,71.01 | 123,71.01 128,71.01 | 128,71.01 133,71.01 | 133,71.01 138,71.01 | T12.1 143,73.76 143,71.41 R4.1 142.1,71.01 138,71.01 | T2.1 93.05,71.06 93,71.01 | T3.1 98.05,71.06 98,71.01 | T5.1 108,73.81 108,71.01 | T6.1 113,73.81 113,71.01 | T7.1 118,73.81 118,71.01 | T8.1 123,73.81 123,71.01 | T9.1 128,73.81 128,71.01 | T10.1 133,73.81 133,71.01 | T11.1 138,73.81 138,71.01 | 113,71.01 116.6,71.01 R5.2 117.4,71.01 118,71.01 | T4.1 103,73.76 103,71.01 | 98,71.01 103,71.01 | 103,71.01 108,71.01 | 93,71.01 91,71.01 88,74.01 88,75.76 T1.1
OEFFNER_1
  Bottom 0.254: X1.A32 153.43,11.91 148,11.91
  Bottom 0.61: 148,11.91 119.6,11.91 115.5,16.01 100,16.01 88.33,27.68 19.33,27.68 16.33,30.68 X2.2
OEFFNER_2  (via drill 0.6)
  Top 0.254: X1.B31 150.89,14.45 148,14.45
  Top 0.61: 148,14.45 121.81,14.45 v120,16.26
  Bottom 0.61: v120,16.26 117.25,19.01 101,19.01 89.56,30.45 20.56,30.45 17.56,33.45 X2.3
OEFFNER_3
  Bottom 0.61: X1.C30 125.29,15.72 119,22.01 102,22.01 86.55,37.46 21.53,37.46 20.03,38.96 X2.5
OEFFNER_4
  Bottom 0.254: X1.A30 153.43,16.99 148,16.99
  Bottom 0.61: 148,16.99 129.52,16.99 121.5,25.01 103,25.01 87.78,40.23 22.78,40.23 21.28,41.73 X2.6
OEFFNER_5  (via drill 0.6)
  Top 0.254: X1.B29 150.89,19.53 148,19.53
  Top 0.61: 148,19.53 131.73,19.53 v127.5,23.76
  Bottom 0.61: v127.5,23.76 123.25,28.01 104,28.01 89.04,42.97 24.04,42.97 22.54,44.47 X2.7
OEFFNER_6
  Bottom 0.61: X1.C28 135.21,20.8 125,31.01 105,31.01 86,50.01 X2.9
OEFFNER_7
  Bottom 0.254: X1.A28 153.43,22.07 148,22.07
  Bottom 0.61: 148,22.07 139.44,22.07 127.5,34.01 106,34.01 87.23,52.78 X2.10
OEFFNER_8  (via drill 0.6)
  Top 0.254: X1.B27 150.89,24.61 148,24.61
  Top 0.61: 148,24.61 141.65,24.61 v135,31.26
  Bottom 0.61: v135,31.26 129.25,37.01 107,37.01 88.46,55.55 X2.11
OEFFNER_9
  Bottom 0.61: X1.C26 145.13,25.88 131,40.01 108,40.01 85.45,62.56 21.55,62.56 20.05,61.06 X2.13
OEFFNER_10
  Bottom 0.254: X1.A26 153.43,27.15 148,27.15
  Bottom 0.61: 148,27.15 145.86,27.15 142.5,30.51 142.5,34.01 133.5,43.01 109,43.01 86.68,65.33 20.32,65.33 18.82,63.83 X2.14
OEFFNER_11  (via drill 0.6)
  Top 0.254: X1.B25 150.89,29.69 148,29.69
  Top 0.61: v142.5,38.76 145.5,35.76 145.5,31.51 147.32,29.69 148,29.69
  Bottom 0.61: v142.5,38.76 135.25,46.01 110,46.01 87.94,68.07 19.06,68.07 17.56,66.57 X2.15
OEFFNER_12
  Bottom 0.61: X1.C24 149.57,31.01 148,31.01 147,32.01 147,39.01 137,49.01 111,49.01 84.9,75.11 18.1,75.11 15.1,72.11 X2.17
OEFFNER_!PF
  Bottom 0.61: X2.1 15.1,27.91 18.08,24.93 42.08,24.93 46,21.01 46,12.67 K1.12
RESET_1
  Top 0.406: X2.19 10.54,32.01 15,32.01
  Top 0.61: 15,32.01 16,32.01 20.06,36.07 C9.1 36.6,34.41 39,32.01 60.28,32.01 D2.2 68,36.01 78,46.01 78,78.51 89,89.51 | 89,89.51 95.75,96.26 142.74,96.26 X1.C1 | T1.3 89,89.51
RESET_2  (via drill 0.6)
  Top 0.406: X2.20 15,34.82
  Top 0.61: 15,34.82 16,34.82 20.05,38.87 C10.1 46.86,38.87 D3.2 53.72,40.01 69,40.01 76,47.01 76,79.76 v90.75,94.51 | T2.3 94,81.51 v107,94.51
  Bottom 0.61: X1.A1 149.57,94.51 v107,94.51 v90.75,94.51
RESET_3  (via drill 0.6)
  Top 0.406: X2.21 15,37.59
  Top 0.61: 15,37.59 16,37.59 20.46,42.05 C11.1 68.04,42.05 74,48.01 74,81.01 v85.75,92.76 D4.2 | X1.C2 143.7,92.76 v110.5,92.76 99,81.26 T3.3
  Bottom 0.61: v85.75,92.76 v110.5,92.76
RESET_4  (via drill 0.6)
  Top 0.406: X2.23 10.59,43.01 15,43.01
  Top 0.61: 15,43.01 16,43.01 21.62,48.63 C12.1 36.6,47.41 39,45.01 60.65,45.01 D5.2 67.63,48.64 72,53.01 72,82.26 v80.75,91.01 | T4.3 104,81.01 v114,91.01
  Bottom 0.254: X1.A2 153.43,88.11 148,88.11
  Bottom 0.61: 148,88.11 145.1,91.01 v114,91.01 v80.75,91.01
RESET_5  (via drill 0.6)
  Top 0.406: X2.24 15,45.87
  Top 0.61: 15,45.87 16,45.87 21.56,51.43 C13.1 46.93,51.43 D6.2 54.09,53.01 68,53.01 70,55.01 70,83.51 v75.75,89.26 | X1.C3 144.6,89.26 v117.5,89.26 109,80.76 T5.3
  Bottom 0.61: v117.5,89.26 v75.75,89.26
RESET_6  (via drill 0.6)
  Top 0.406: X2.25 15,48.61
  Top 0.61: 15,48.61 16,48.61 22,54.61 C14.1 66.6,54.61 68,56.01 68,84.76 v70.75,87.51 69,89.26 D7.2 | T6.3 114,80.51 v121,87.51
  Bottom 0.254: X1.A3 153.43,85.57 148,85.57
  Bottom 0.61: 148,85.57 146.06,87.51 v121,87.51 v70.75,87.51
RESET_7  (via drill 0.6)
  Top 0.406: X2.27 15,54.15
  Top 0.61: 15,54.15 16,54.15 23.03,61.18 C15.1 36.6,59.41 39,57.01 60.11,57.01 D8.2 64.28,61.29 66,63.01 v66,85.76 | X1.C4 145.62,85.76 v124.5,85.76 119,80.26 T7.3
  Bottom 0.61: v66,85.76 v124.5,85.76
RESET_8  (via drill 0.6)
  Top 0.406: X2.28 15,56.92
  Top 0.61: 15,56.92 16,56.92 23.06,63.98 C16.1 46.92,63.98 D9.2 64,75.46 v64,84.01 | T8.3 124,80.01 v128,84.01
  Bottom 0.254: X1.A4 153.43,83.03 148,83.03
  Bottom 0.61: 148,83.03 147.02,84.01 v128,84.01 v64,84.01
RESET_9  (via drill 0.6)
  Top 0.406: X2.29 15,59.69
  Top 0.61: 15,59.69 16,59.69 23.46,67.15 C17.1 D10.2 52.14,67.15 62,77.01 v62,82.26 | T9.3 129,79.76 v131.5,82.26
  Bottom 0.254: X1.B5 150.89,80.49 148,80.49
  Bottom 0.61: 148,80.49 146.23,82.26 v131.5,82.26 v62,82.26
RESET_10  (via drill 0.6)
  Top 0.406: X2.31 15,65.2
  Top 0.61: 15,65.2 16,65.2 25,74.2 25,77.01 27.4,79.41 C18.1 D11.2 | D11.2 | v49,79.41 D11.2 | T10.3 134,79.51 v135,80.51
  Bottom 0.254: X1.B6 150.89,77.95 148,77.95
  Bottom 0.61: 148,77.95 145.44,80.51 v135,80.51 50.1,80.51 v49,79.41
RESET_11  (via drill 0.6)
  Top 0.406: X2.32 15,67.97
  Top 0.61: 15,67.97 16,67.97 23,74.97 23,80.01 26.2,83.21 C19.1 37.2,83.21 40,86.01 | D12.2 40,86.01 | 40,86.01 43.75,82.26 50.5,82.26 v54,78.76 | T11.3 139,78.26 v138.5,78.76
  Bottom 0.254: X1.B7 150.89,75.41 148,75.41
  Bottom 0.61: 148,75.41 144.65,78.76 v138.5,78.76 v54,78.76
RESET_12  (via drill 0.6)
  Top 0.406: X2.33 15,70.71
  Top 0.61: 15,70.71 16,70.71 21,75.71 21,82.01 25,86.01 C20.1 26.6,87.61 29,90.01 50.28,90.01 D13.2 54.28,81.73 v59,77.01 | T12.3 143.2,77.01 v142,77.01
  Bottom 0.254: X1.B8 150.89,72.87 148,72.87
  Bottom 0.61: v59,77.01 v142,77.01 143.86,77.01 148,72.87
RESET_ALL
  Top 0.406: X2.18 15,29.31
  Top 0.61: R7.2 91.25,68.76 84.9,75.11 82.1,75.11 80,73.01 80,45.01 64.3,29.31 C21.1 15,29.31
SCL
  Bottom 0.254: X1.B18 150.89,44.93 148,44.93
  Bottom 0.61: X1.C20 147.5,43.24 147.5,44.43 148,44.93
SDA
  Bottom 0.254: X1.B17 150.89,47.47 148,47.47
  Bottom 0.61: X1.C21 146,42.2 146,45.47 148,47.47
V+  (via drill 0.6)  (1 unrouted)
  Top 0.406: X2.30 15,62.43 | X2.22 15,40.33 | 15,51.41 X2.26
  Top 0.61: 15,62.43 16,62.43 23.52,69.95 v25,69.95 C8.1 | 15,51.41 16,51.41 22.01,57.42 v25,57.42 C7.1 | C6.1 v25,44.85 20.52,44.85 16,40.33 15,40.33 | v25,32.33 C5.1 | 145,73.81 T12.2 145,73.76 v145,72.76 145,71.41 R4.2 | T2.2 95,73.76 v95,72.76 | T3.2 100,73.76 v100,72.76 | T4.2 105,73.76 v105,72.76 | T5.2 110,73.76 v110,72.76 | T6.2 115,73.76 v115,72.76 | T7.2 120,73.76 v120,72.76 | T8.2 125,73.76 v125,72.76 | T9.2 130,73.76 v130,72.76 | T10.2 135,73.76 v135,72.76 | T11.2 140,73.76 v140,72.76 | T1.2 90,75.76 v90,74.76
  Top 0.813: v84,6.36 80.79,6.36 79.52,7.63 IC1.2 | v85,69.95 93.51,61.44 89.02,61.44 v85,57.42 | 97.52,44.85 v85,44.85 | v84,10.8 84,31.33 v85,32.33
  Top 1.93: F1.1 C2.1 C1.+ 114.11,61.44 | 114.11,61.44 93.51,61.44 | v85,32.33 114.11,61.44
  Bottom 0.406: X2.37 X2.4 | X2.45 X2.12 | X2.49 X2.16 | X2.8 X2.41
  Bottom 0.61: X2.4 18.82,36.19 22.68,32.33 v25,32.33 v85,32.33 | X2.16 16.33,69.34 16.94,69.95 v25,69.95 v85,69.95 | X2.12 21.28,58.29 22.15,57.42 v25,57.42 v85,57.42 | v85,44.85 v25,44.85 24.16,44.85 21.77,47.24 X2.8
  Bottom 0.813: v84,10.8 v84,6.36
  Bottom 1.016: v145,72.76 v140,72.76 v135,72.76 v130,72.76 v125,72.76 v120,72.76 v115,72.76 v110,72.76 v105,72.76 v100,72.76 v95,72.76 92,72.76 v90,74.76
  Bottom 1.93: v120,72.76 120,61.44 C1.+
WECHSLER_1  (via drill 0.6)
  Top 0.254: X1.B32 150.89,11.91 148,11.91
  Top 0.61: 148,11.91 116.85,11.91 v116.25,12.51
  Bottom 0.406: X2.35 11.23,30.68 12.6,29.31 15,29.31
  Bottom 0.61: v116.25,12.51 114.25,14.51 99.5,14.51 87.7,26.31 18.7,26.31 15.7,29.31 15,29.31
WECHSLER_2
  Bottom 0.406: X2.36 11.21,33.45 12.59,32.07 15,32.07
  Bottom 0.61: X1.C31 120.33,13.18 116,17.51 100.5,17.51 88.94,29.07 19.94,29.07 16.94,32.07 15,32.07
WECHSLER_3
  Bottom 0.254: X1.A31 153.43,14.45 148,14.45
  Bottom 0.406: X2.38 11.23,38.96 12.61,37.58 15,37.58
  Bottom 0.61: 148,14.45 124.56,14.45 118.5,20.51 101.5,20.51 85.93,36.08 20.93,36.08 19.43,37.58 15,37.58
WECHSLER_4  (via drill 0.6)
  Top 0.254: X1.B30 150.89,16.99 148,16.99
  Top 0.61: 148,16.99 126.77,16.99 v123.75,20.01
  Bottom 0.406: X2.39 11.23,41.73 12.63,40.33 15,40.33
  Bottom 0.61: v123.75,20.01 120.25,23.51 102.5,23.51 87.18,38.83 22.18,38.83 20.68,40.33 15,40.33
WECHSLER_5
  Bottom 0.406: X2.40 11.23,44.47 12.6,43.1 15,43.1
  Bottom 0.61: X1.C29 130.25,18.26 122,26.51 103.5,26.51 88.41,41.6 23.41,41.6 21.91,43.1 15,43.1
WECHSLER_6
  Bottom 0.254: X1.A29 153.43,19.53 148,19.53
  Bottom 0.406: X2.42 11.22,50.01 12.61,48.62 15,48.62
  Bottom 0.61: 148,19.53 134.48,19.53 124.5,29.51 104.5,29.51 85.39,48.62 15,48.62
WECHSLER_7  (via drill 0.6)
  Top 0.254: X1.B28 150.89,22.07 148,22.07
  Top 0.61: 148,22.07 136.69,22.07 v131.25,27.51
  Bottom 0.406: X2.43 11.23,52.78 12.6,51.41 15,51.41
  Bottom 0.61: v131.25,27.51 126.25,32.51 105.5,32.51 86.6,51.41 15,51.41
WECHSLER_8
  Bottom 0.406: X2.44 11.21,55.55 12.59,54.17 15,54.17
  Bottom 0.61: X1.C27 140.17,23.34 128,35.51 106.5,35.51 87.84,54.17 15,54.17
WECHSLER_9
  Bottom 0.254: X1.A27 153.43,24.61 148,24.61
  Bottom 0.406: X2.46 11.23,61.06 12.62,59.67 15,59.67
  Bottom 0.61: 148,24.61 144.4,24.61 130.5,38.51 107.5,38.51 84.84,61.17 22.16,61.17 20.66,59.67 15,59.67
WECHSLER_10  (via drill 0.6)
  Top 0.254: X1.B26 150.89,27.15 148,27.15
  Top 0.61: 148,27.15 146.61,27.15 v138.75,35.01
  Bottom 0.406: X2.47 11.22,63.83 12.62,62.43 15,62.43
  Bottom 0.61: v138.75,35.01 132.25,41.51 108.5,41.51 86.08,63.93 20.92,63.93 19.42,62.43 15,62.43
WECHSLER_11
  Bottom 0.406: 15,65.2 12.6,65.2 11.23,66.57 X2.48
  Bottom 0.61: X1.C25 146.59,28.42 144,31.01 144,34.51 134,44.51 109.5,44.51 87.31,66.7 19.69,66.7 18.19,65.2 15,65.2
WECHSLER_12
  Bottom 0.254: X1.A25 153.43,29.69 148,29.69
  Bottom 0.406: X2.50 11.22,72.11 12.61,70.72 15,70.72
  Bottom 0.61: 148,29.69 147.32,29.69 145.5,31.51 145.5,38.51 136.5,47.51 110.5,47.51 84.29,73.72 18.71,73.72 15.71,70.72 15,70.72
WECHSLER_!PF  (via drill 0.6)
  Top 0.61: K1.7 48.19,23.18 v41,23.18
  Bottom 0.61: v41,23.18 12.39,23.18 X2.34

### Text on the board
Top: Top | Rev. 1.1 | Absorberüberwachung Interface 2015-08-15 MH
Bottom: Bottom
tPlace: D4 | D7 | C20 | C19 | D12 | D13 | T1 | T12 | C18 | T2 | T3 | T4 | T5 | T6 | T7 | T8 | T9 | T10 | T11 | D11 | C8 | T13 | R5 | D10 | R4 | C17 | R7 | C15 | R6 | C16 | Reset ALL | D9 | D8 | C2 | F1 | C14 | C7 | C1 | C12 | C13 | D6 | D5 | C11 | C6 | C9 | C10 | D3 | D2 | C21 | C5 | C4 | R2 | datacrumbs | R3 | R1 | K1 | C3 | IC1
bPlace: 1 | 2 | 3 | 4 | 5 | 6 | 7 | 8 | 9 | 10 | 11 | 12 | 13 | 14 | 15 | 16 | 17 | 18 | 33 | 34 | 35 | 36 | 37 | 38 | 39 | 40 | 41 | 42 | 43 | 44 | 45 | 46 | 47 | 48 | 49 | 50 | +Ub | 30 | Öffner 9 | 13 | Öffner !PF | 1 | Reset 10 | 31 | Öffner 10 | 14 | Öffner 1 | 2 | Reset 11 | 32 | Öffner 11 | 15 | Öffner 2 | 3 | Reset 12 | 33 | +Ub | 16 | +Ub | 4 | Wechsler !PF | 34 | Öffner 12 | 17 | Öffner 3 | 5 | Wechsler 1 | 35 | Reset ALL | 18 | Öffner 4 | 6 | Wechsler 2 | 36 | Reset 1 | 19 | Öffner 5 | 7 | +Ub | 37 | Reset 2 | 20 | +Ub | 8 | Wechsler 3 | 38 | Reset 3 | 21 | Öffner 6 | 9 | Wechsler 4 | 39 | +Ub | 22 | Öffner 7 | 10 | Wechsler 5 | 40 | Reset 4 | 23 | Öffner 8 | 11 | +Ub | 41 | Reset 5 | 24 | +Ub | 12 | Wechsler 6 | 42 | Reset 6 | 25 | Wechsler 7 | 43 | +Ub | 26 | Wechsler 8 | 44 | Reset 7 | 27 | +Ub | 45 | Reset 8 | 28 | Wechsler 9 | 46 | Reset 9 | 29 | Wechsler 10 | 47 | Wechsler 11 | 48 | D1 | +Ub | 49 | Wechsler 12 | 50 | datacrumbs
DrillLegend: LAYER-STACK
DrillLegend_01-16: 01-16
DrillLegend_01-20: 01-20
